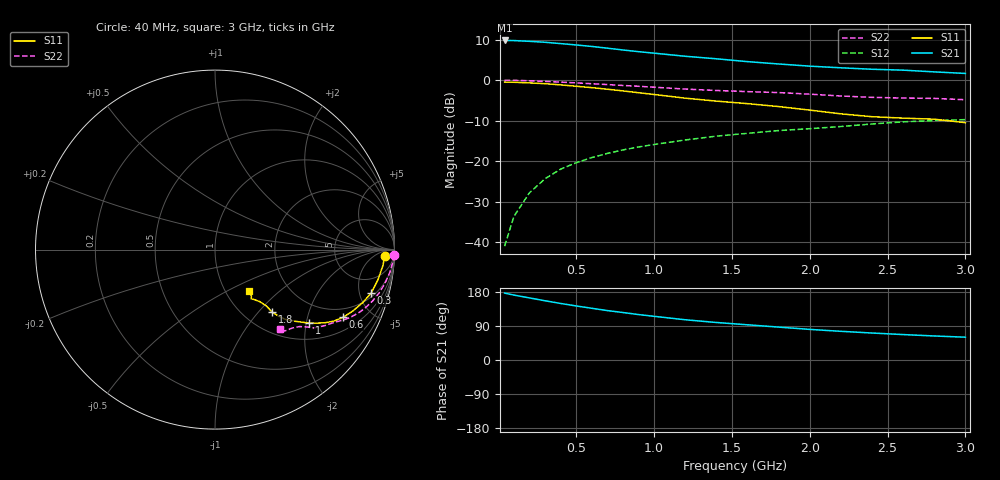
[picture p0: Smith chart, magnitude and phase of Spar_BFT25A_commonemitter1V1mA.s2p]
! Filename:  BFT25AD.S2P  Version:  2.0
! NXP part #: BFT25A  Date: Aug 1990
! Bias condition: Vce=1V, Ic=1mA
#  MHz  S  MA  R  50
! Freq  S11  S21  S12  S22  !GUM [dB]
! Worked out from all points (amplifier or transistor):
!   21 points, 40 MHz to 3 GHz, reference 50 ohm
!   highest |S21| = 9.8 dB at 40 MHz (marker M1)
!   |S21| within 3 dB of that: start of sweep to 965 MHz
!   unconditionally stable (mu >= 1): 2.046 GHz to end of sweep
!   at 300 MHz: K = 0.23, MSG = 16.8 dB, |S12| = -24.3 dB
!   at 1 GHz: K = 0.65, MSG = 11.3 dB, |S12| = -15.9 dB
!   at 3 GHz: K = 1.12, MAG = 3.6 dB, |S12| = -9.7 dB
!   S11 on the Smith chart (normalised r, x): 40 MHz: 24, -17; 300 MHz: 2.43, -6.40; 600 MHz: 1.55, -3.36; 1 GHz: 1.42, -2.08; 1.8 GHz: 1.33, -1.19; 3 GHz: 1.29, -0.65
40  0.946 -2.2  3.078 176.5  0.009 86.5  0.996 -1.6
100  0.94 -5.4  3.067 171.3  0.021 85.3  0.993 -4.0
200  0.923 -10.6  3.003 163.8  0.041 82.7  0.981 -7.8
300  0.903 -15.6  2.923 156.3  0.061 79.5  0.964 -11.5
400  0.873 -19.9  2.815 149.2  0.08 76.7  0.945 -14.9
500  0.84 -24.1  2.708 142.6  0.096 74.5  0.924 -18.0
600  0.807 -27.9  2.597 136.5  0.111 72.2  0.902 -20.7
700  0.772 -31.1  2.472 130.4  0.125 70.0  0.881 -23.1
800  0.736 -33.6  2.35 125.3  0.138 68.5  0.859 -25.1
900  0.699 -35.9  2.24 119.9  0.15 67.0  0.839 -27.0
1000  0.665 -38.0  2.147 115.3  0.161 65.6  0.817 -28.6
1200  0.599 -41.8  1.966 106.2  0.183 63.0  0.775 -31.7
1400  0.551 -44.8  1.83 99.0  0.204 61.2  0.745 -34.6
1600  0.513 -46.3  1.688 92.9  0.221 60.2  0.721 -36.7
1800  0.472 -47.6  1.58 86.8  0.239 59.0  0.702 -38.4
2000  0.427 -47.6  1.485 80.8  0.252 57.1  0.671 -40.0
2200  0.384 -49.2  1.417 75.7  0.268 55.4  0.637 -42.3
2400  0.354 -51.8  1.36 71.2  0.288 54.2  0.613 -45.5
2600  0.34 -53.7  1.326 67.1  0.306 52.9  0.601 -48.5
2800  0.33 -52.0  1.262 63.4  0.317 52.2  0.595 -49.7
3000  0.299 -50.0  1.208 60.2  0.326 51.6  0.573 -50.7
